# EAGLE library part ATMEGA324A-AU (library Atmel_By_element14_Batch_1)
8-bit Atmel Microcontroller
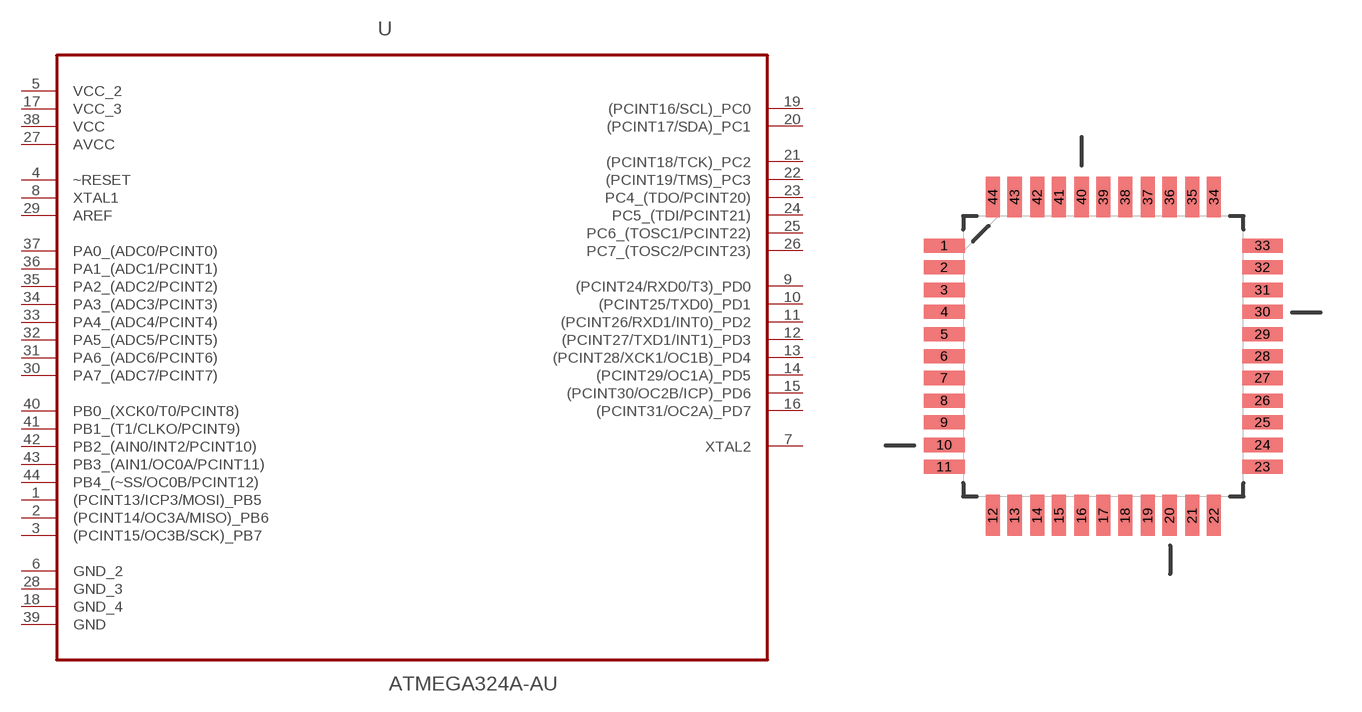
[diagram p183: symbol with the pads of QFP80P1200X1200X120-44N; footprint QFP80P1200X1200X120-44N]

Designator prefix U

## ATMEGA324A-AU (DESCRIPTION: 8-bit Atmel Microcontroller; MPN: ATMEGA324A-AU; OC_FARNELL: 1841608; OC_NEWARK: 12T1299; PACKAGE: QFP-44; SUPPLIER: Atmel)  [QFP80P1200X1200X120-44N]
1  (PCINT13/ICP3/MOSI)_PB5
2  (PCINT14/OC3A/MISO)_PB6
3  (PCINT15/OC3B/SCK)_PB7
4  ~RESET  in
5  VCC_2  pwr
6  GND_2  pas
7  XTAL2  out
8  XTAL1  in
9  (PCINT24/RXD0/T3)_PD0
10  (PCINT25/TXD0)_PD1
11  (PCINT26/RXD1/INT0)_PD2
12  (PCINT27/TXD1/INT1)_PD3
13  (PCINT28/XCK1/OC1B)_PD4
14  (PCINT29/OC1A)_PD5
15  (PCINT30/OC2B/ICP)_PD6
16  (PCINT31/OC2A)_PD7
17  VCC_3  pwr
18  GND_4  pas
19  (PCINT16/SCL)_PC0
20  (PCINT17/SDA)_PC1
21  (PCINT18/TCK)_PC2
22  (PCINT19/TMS)_PC3
23  PC4_(TDO/PCINT20)
24  PC5_(TDI/PCINT21)
25  PC6_(TOSC1/PCINT22)
26  PC7_(TOSC2/PCINT23)
27  AVCC  pwr
28  GND_3  pas
29  AREF  in
30  PA7_(ADC7/PCINT7)
31  PA6_(ADC6/PCINT6)
32  PA5_(ADC5/PCINT5)
33  PA4_(ADC4/PCINT4)
34  PA3_(ADC3/PCINT3)
35  PA2_(ADC2/PCINT2)
36  PA1_(ADC1/PCINT1)
37  PA0_(ADC0/PCINT0)
38  VCC  pwr
39  GND  pas
40  PB0_(XCK0/T0/PCINT8)
41  PB1_(T1/CLKO/PCINT9)
42  PB2_(AIN0/INT2/PCINT10)
43  PB3_(AIN1/OC0A/PCINT11)
44  PB4_(~SS/OC0B/PCINT12)

## Footprint QFP80P1200X1200X120-44N (pad centres in mm)
smd 1.473 x 0.508: 1 -5.74,3.988; 2 -5.74,3.2; 3 -5.74,2.388; 4 -5.74,1.6; 5 -5.74,0.787; 6 -5.74,0; 7 -5.74,-0.787; 8 -5.74,-1.6; 9 -5.74,-2.388; 10 -5.74,-3.2; 11 -5.74,-3.988; 23 5.74,-3.988; 24 5.74,-3.2; 25 5.74,-2.388; 26 5.74,-1.6; 27 5.74,-0.787; 28 5.74,0; 29 5.74,0.787; 30 5.74,1.6; 31 5.74,2.388; 32 5.74,3.2; 33 5.74,3.988
smd 0.508 x 1.473: 12 -3.988,-5.74; 13 -3.2,-5.74; 14 -2.388,-5.74; 15 -1.6,-5.74; 16 -0.787,-5.74; 17 0,-5.74; 18 0.787,-5.74; 19 1.6,-5.74; 20 2.388,-5.74; 21 3.2,-5.74; 22 3.988,-5.74; 34 3.988,5.74; 35 3.2,5.74; 36 2.388,5.74; 37 1.6,5.74; 38 0.787,5.74; 39 0,5.74; 40 -0.787,5.74; 41 -1.6,5.74; 42 -2.388,5.74; 43 -3.2,5.74; 44 -3.988,5.74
